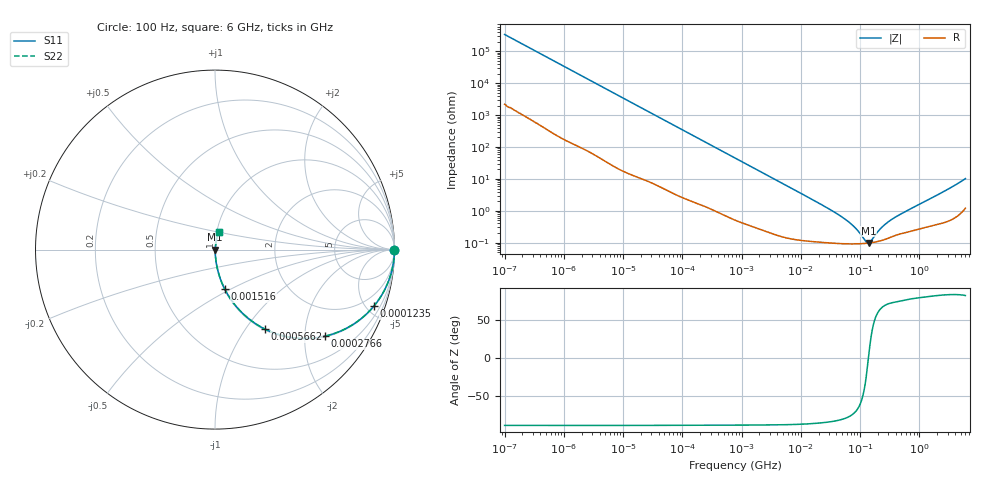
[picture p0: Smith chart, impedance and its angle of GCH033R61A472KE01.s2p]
!Murata Part Number: GCH033R61A472KE01
!These Parameters are Measured in Series Mode Connection
!Data Generated on Jun 19, 2026
!  o--ll--o
!Port1  Port2
!  o------o
!Operation Temp=25[degC], DC Bias Voltage=0[V]
!Freq. Start=100[Hz] Stop=6[GHz] 401[Steps]
# Hz S RI R 50
!Freq.(Hz) S11(Real) S11(Imag) S21(Real) S21(Imag) S12(Real) S12(Imag) S22(Real) S22(Imag)
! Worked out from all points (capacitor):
!   401 points, 100 Hz to 6 GHz, reference 50 ohm
!   read as one part in series: C = 4.71 nF near 109 Hz
!   lowest |Z| = 97.5 mohm at 139.6 MHz (marker M1)
!   series resonance near 138.4 MHz, so ESL is about 280 pH
!   S11 on the Smith chart (normalised r, x): 100 Hz: open; 123.5 kHz: 1.04, -5.60; 276.6 kHz: 1.02, -2.51; 566.2 kHz: 1.01, -1.23; 1.516 MHz: 1.01, -0.46; 6 GHz: 1.02, +0.20
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100  1 -0.000296  2e-06 0.000296  2e-06 0.000296  1 -0.000296
2008  0.9999 -0.00589  6.66e-05 0.00589  6.66e-05 0.00589  0.9999 -0.00589
12592  0.9985 -0.0366  0.00154 0.0366  0.00154 0.0366  0.9985 -0.0366
40335  0.9857 -0.1153  0.0143 0.1153  0.0143 0.1153  0.9857 -0.1153
123542  0.8851 -0.315  0.1149 0.315  0.1149 0.315  0.8851 -0.315
184852  0.7768 -0.412  0.2232 0.412  0.2232 0.412  0.7768 -0.412
276587  0.6115 -0.4826  0.3885 0.4826  0.3885 0.4826  0.6115 -0.4826
395726  0.4375 -0.491  0.5625 0.491  0.5625 0.491  0.4375 -0.491
566185  0.2778 -0.4426  0.7222 0.4426  0.7222 0.4426  0.2778 -0.4426
774597  0.1723 -0.372  0.8277 0.372  0.8277 0.372  0.1723 -0.372
1516199  0.0537 -0.2186  0.9463 0.2186  0.9463 0.2186  0.0537 -0.2186
4060267  0.00917 -0.0861  0.9908 0.0861  0.9908 0.0861  0.00917 -0.0861
1.555665e7  0.00159 -0.0226  0.9984 0.0226  0.9984 0.0226  0.00159 -0.0226
5.960426e7  0.000942 -0.00491  0.9991 0.00491  0.9991 0.00491  0.000942 -0.00491
8.527865e7  0.000924 -0.00261  0.9991 0.00261  0.9991 0.00261  0.000924 -0.00261
1.220122e8  0.00095 -0.000654  0.9991 0.000654  0.9991 0.000654  0.00095 -0.000654
1.395531e8  0.000973 4.46e-05  0.999 -4.46e-05  0.999 -4.46e-05  0.000973 4.46e-05
1.526266e8  0.000995 0.000509  0.999 -0.000509  0.999 -0.000509  0.000995 0.000509
2.283698e8  0.00117 0.00268  0.9988 -0.00268  0.9988 -0.00268  0.00117 0.00268
3.124326e8  0.00144 0.00455  0.9986 -0.00455  0.9986 -0.00455  0.00144 0.00455
2.048624e9  0.0047 0.0314  0.9953 -0.0314  0.9953 -0.0314  0.0047 0.0314
6e9  0.0217 0.098  0.9783 -0.098  0.9783 -0.098  0.0217 0.098
